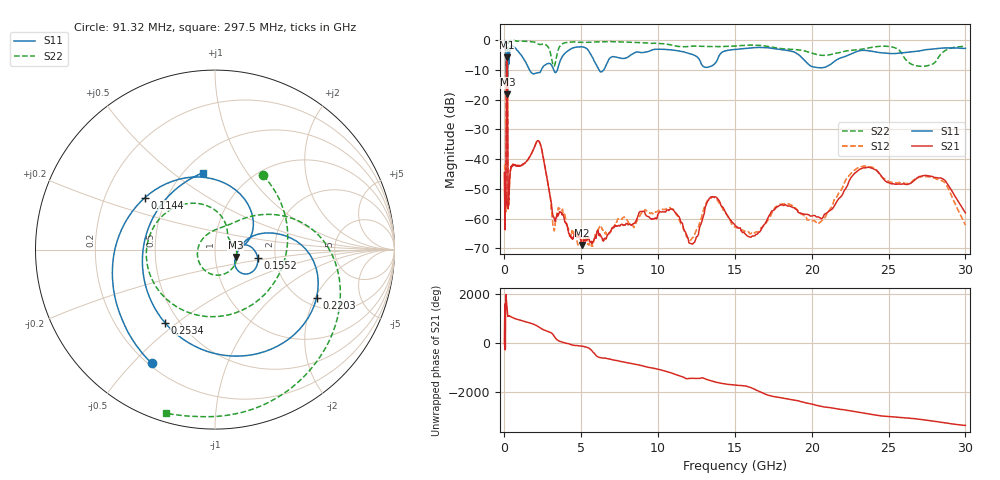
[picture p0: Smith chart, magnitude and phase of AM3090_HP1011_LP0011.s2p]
! Date/Time: Thu, Feb 28, 2019 2:05 PM
! Network Analyzer: Agilent Technologies E8364B Rev: A.07.50.67
! Sweep from 0.010 to 30.000 GHz, 1601 Points, Sweep Type: LOG
! Power Supply: 5.023 V, 0.002 A
# Hz S DB R 50
!freq MagS11 AngS11 MagS21 AngS21 MagS12 AngS12 MagS22 AngS22
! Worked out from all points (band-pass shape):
!   1601 points, 10 MHz to 30 GHz, reference 50 ohm
!   highest |S21| = -5.77 dB at 157.6 MHz (marker M1); lowest = -68.9 dB at 5.052 GHz (marker M2)
!   |S21| within 3 dB of the highest: 129.5 MHz to 191.8 MHz (62.34 MHz wide, 38.8 % of centre)
!   lowest |S11| = -18.3 dB at 186.8 MHz (marker M3), VSWR 1.28, Z = 62.7 - j5.18 ohm
!   |S11| at or under -10 dB: 1.624 GHz to 2.4 GHz (776.3 MHz wide, 38.6 % of centre); 3.203 GHz to 3.447 GHz (243.7 MHz wide, 7.33 % of centre); 6.145 GHz to 6.468 GHz (322.2 MHz wide, 5.11 % of centre)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
!   |S22| runs from -20.8 to -0.2 dB; largest |S21 - S12| = 0.013
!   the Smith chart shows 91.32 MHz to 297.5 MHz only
!   S11 on the Smith chart (normalised r, x): 91.32 MHz: 0.21, -0.57; 114.4 MHz: 0.38, +0.29; 155.2 MHz: 1.61, -0.15; 220.3 MHz: 2.33, -2.06; 253.4 MHz: 0.42, -0.45; 297.5 MHz: 0.62, +0.65
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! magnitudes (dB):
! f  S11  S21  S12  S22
! 10 MHz  -0.2  -44.6  -41.8  -0.5
! 38.04 MHz  -0.4  -60.8  -59.7  -1.3
! 49.1 MHz  -0.7  -51.1  -48.9  -1.4
! 91.32 MHz  -2.8  -55.3  -56.9  -6.1
! 114.4 MHz  -6.3  -23.5  -23.5  -8.2
! 144.7 MHz  -14.6  -6.0  -6.0  -19.6
! 155.2 MHz  -12.3  -5.8  -5.7  -17.1
! 157.6 MHz  -12.1  -5.8  -5.7  -16.9
! 186.8 MHz  -18.3  -7.6  -7.6  -19.6
! 220.3 MHz  -4.1  -44.2  -44.0  -2.8
! 253.4 MHz  -6.1  -55.1  -54.7  -0.8
! 297.5 MHz  -7.3  -51.9  -52.9  -0.4
! 550.5 MHz  -2.0  -41.7  -42.0  -0.2
! 2.084 GHz  -11.1  -34.3  -34.2  -1.0
! 3.204 GHz  -10.0  -59.5  -63.2  -8.8
! 5.052 GHz  -2.3  -68.9  -67.1  -0.8
! 7.926 GHz  -6.0  -61.6  -60.2  -0.7
! 12.19 GHz  -4.8  -68.4  -66.7  -2.1
! 13.68 GHz  -8.0  -52.7  -52.9  -2.2
! 16.13 GHz  -2.6  -65.8  -64.6  -1.7
! 23.48 GHz  -3.5  -43.0  -42.4  -2.9
! 30 GHz  -2.8  -58.1  -62.2  -2.2
